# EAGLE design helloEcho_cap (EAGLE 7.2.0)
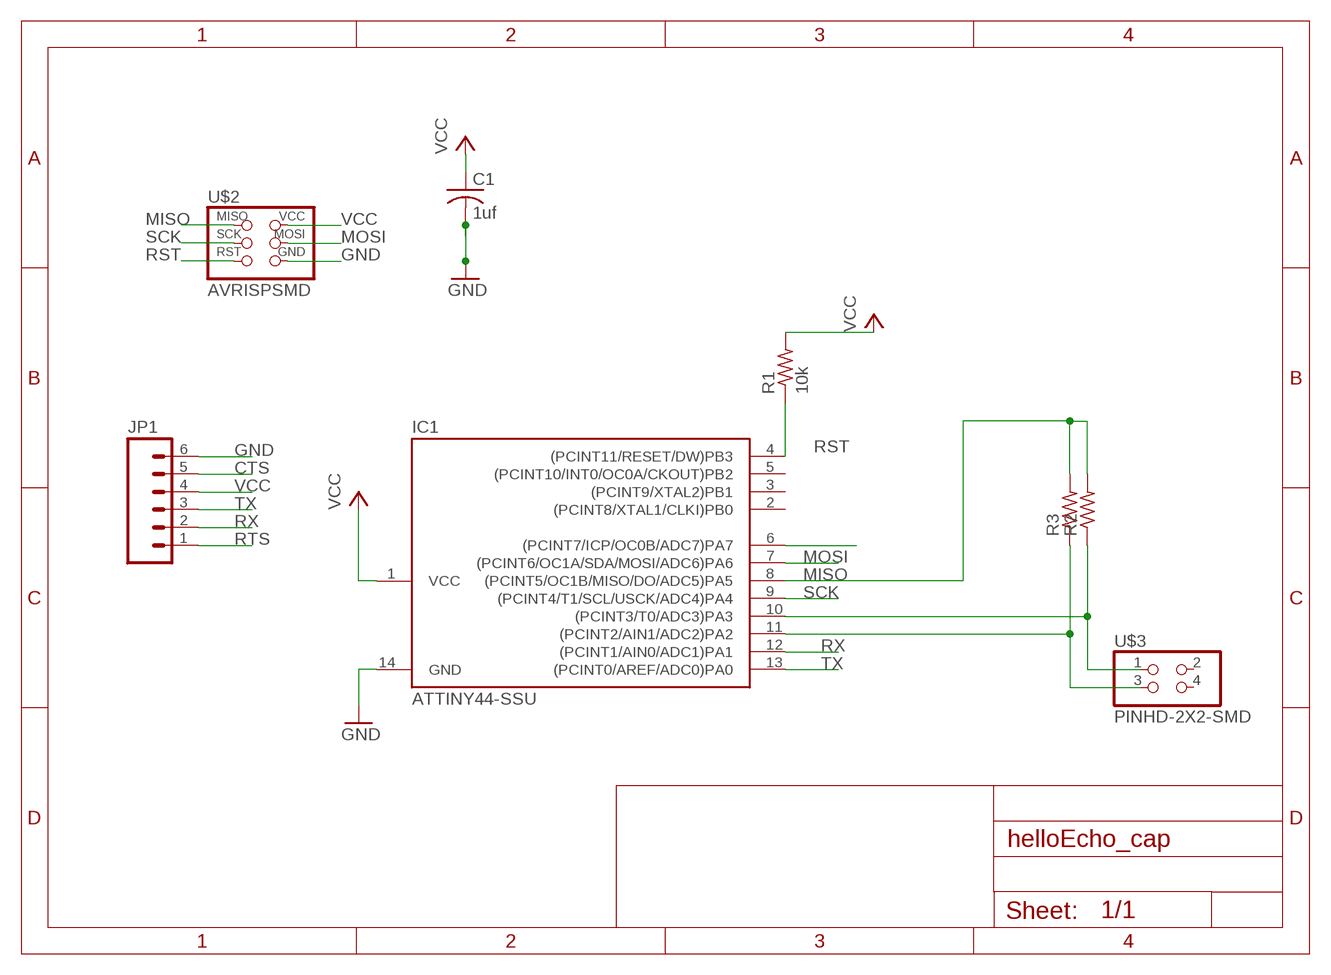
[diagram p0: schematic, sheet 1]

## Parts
C1  1uf  C-USC1206  [C1206]
IC1  ATTINY44-SSU  [SOIC14]
JP1  M06SMD  [1X06-SMD]
R1  10k  R-US_R1206  [R1206]
R2  RESISTOR1206  [1206]
R3  RESISTOR1206  [1206]
U$2  AVRISPSMD  [2X03SMD]
U$3  PINHD-2X2-SMD  [2X02SMD]

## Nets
CTS: JP1.5
GND: C1.2 IC1.14(GND) JP1.6 U$2.6(GND)
MISO: IC1.8((PCINT5/OC1B/MISO/DO/ADC5)PA5) R2.2 R3.2 U$2.1(MISO)
MOSI: IC1.7((PCINT6/OC1A/SDA/MOSI/ADC6)PA6) U$2.4(MOSI)
N$3: IC1.6((PCINT7/ICP/OC0B/ADC7)PA7)
N$5: IC1.10((PCINT3/T0/ADC3)PA3) R2.1 U$3.1
N$6: IC1.11((PCINT2/AIN1/ADC2)PA2) R3.1 U$3.3
RST: IC1.4((PCINT11/RESET/DW)PB3) R1.1 U$2.5(RST)
RTS: JP1.1
RX: IC1.12((PCINT1/AIN0/ADC1)PA1) JP1.2
SCK: IC1.9((PCINT4/T1/SCL/USCK/ADC4)PA4) U$2.3(SCK)
TX: IC1.13((PCINT0/AREF/ADC0)PA0) JP1.3
VCC: C1.1 IC1.1(VCC) JP1.4 R1.2 U$2.2(VCC)
Unconnected: IC1.2((PCINT8/XTAL1/CLKI)PB0) IC1.3((PCINT9/XTAL2)PB1) IC1.5((PCINT10/INT0/OC0A/CKOUT)PB2) U$3.2 U$3.4

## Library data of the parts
C1 = rcl:C-US: CAPACITOR, American symbol
IC1 = fab:ATTINY44
JP1 = SparkFun:M06: Header 6 Standard 6-pin 0.1" header. Use with straight break away headers (SKU : PRT-00116), right angle break away headers (PRT-00553), swiss pins (PRT-00743), machine pins (PRT-00117), and female headers (PRT-00115). Molex polarized connector foot print use with SKU : PRT-08094 with associated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
R1 = resistor:R-US_: RESISTOR, American symbol
R2 R3 = 01_FAB_Hello:RESISTOR
U$2 = fab:AVRISP
U$3 = 01_fab:PINHD-2X2-SMD

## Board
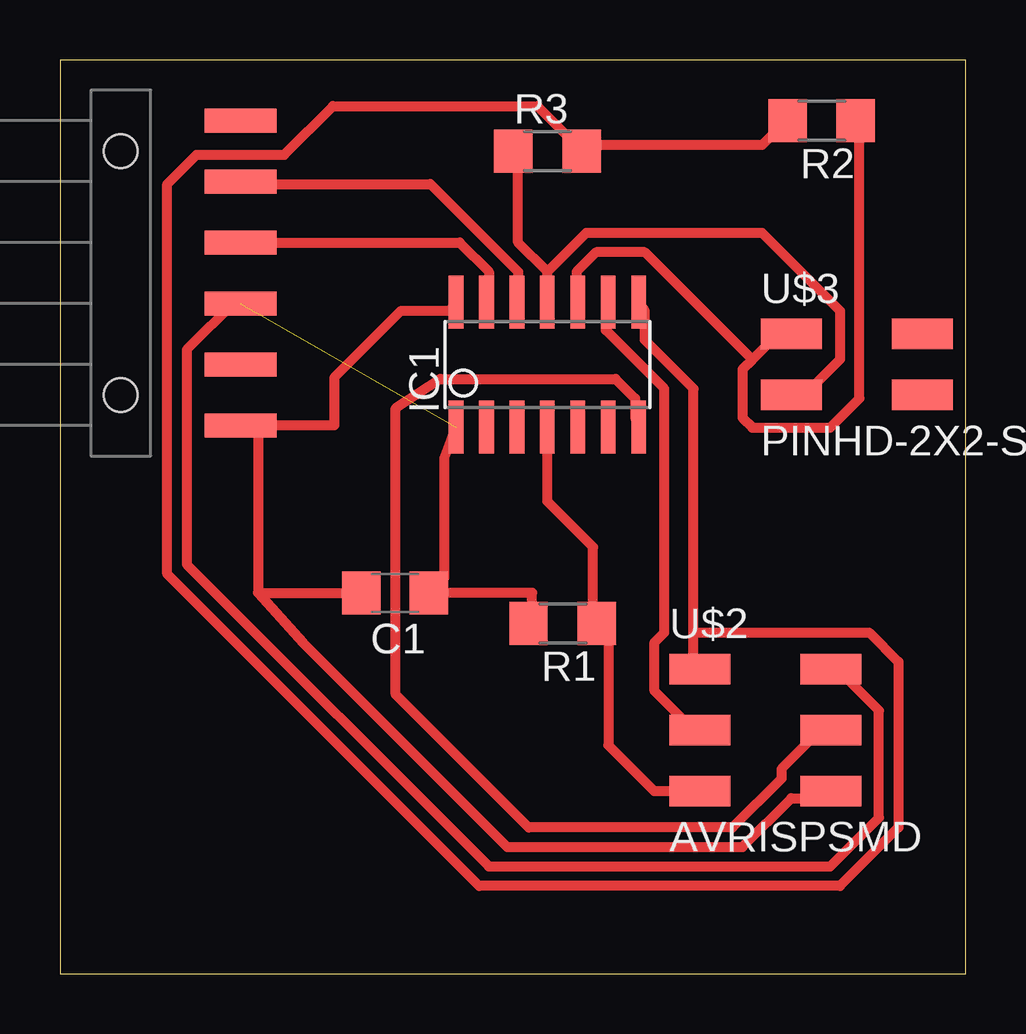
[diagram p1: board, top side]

Size 37.77 x 38.09 mm. Coordinates in mm from the lower left corner, seen from the top.
Outline: 0,0 37.77,0 37.77,38.09 0,38.09 0,0
Copper layers (1*16): Top 0.035mm / dielectric 1.5mm / Bottom 0.035mm
Design rules "default *": minimum track width 16mil, minimum drill 24mil, track to track 16mil, track to pad 16mil, pad to pad 16mil, via to via 16mil, smd to smd 16mil, copper to edge 40mil, drill to drill 8mil, minimum pad ring 10mil, minimum via ring 8mil, stop-mask expansion 4mil, vias tented up to drill 0mil, thermal gap 10mil

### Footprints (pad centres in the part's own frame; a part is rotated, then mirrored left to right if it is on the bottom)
C1206 = smd 1.6 x 1.8: 1 -1.4,0; 2 1.4,0
SOIC14 = smd 0.61 x 2.21: 1 -3.81,-2.603; 2 -2.54,-2.603; 3 -1.27,-2.603; 4 0,-2.603; 5 1.27,-2.603; 6 2.54,-2.603; 7 3.81,-2.603; 8 3.81,2.603; 9 2.54,2.603; 10 1.27,2.603; 11 0,2.603; 12 -1.27,2.603; 13 -2.54,2.603; 14 -3.81,2.603
1X06-SMD = smd 1 x 3: 1 -6.35,5; 2 -3.81,5; 3 -1.27,5; 4 1.27,5; 5 3.81,5; 6 6.35,5 | hole 1.4: -5.08,0; 5.08,0
R1206 = smd 1.6 x 1.803: 1 -1.422,0; 2 1.422,0
1206 = smd 1.6 x 1.803: 1 -1.422,0; 2 1.422,0
2X03SMD = smd 2.54 x 1.27: 1 -2.54,2.54; 2 2.92,2.54; 3 -2.54,0; 4 2.92,0; 5 -2.54,-2.54; 6 2.92,-2.54
2X02SMD = smd 2.54 x 1.27: 1 -2.54,1.27; 2 2.92,1.27; 3 -2.54,-1.27; 4 2.92,-1.27

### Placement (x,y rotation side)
C1  13.97,15.88 180 top
IC1  20.32,25.4 0 top
JP1  2.54,29.21 270 top
R1  20.95,14.61 180 top
R2  31.75,35.56 180 top
R3  20.32,34.29 0 top
U$2  29.21,10.16 0 top
U$3  33.02,25.4 0 top

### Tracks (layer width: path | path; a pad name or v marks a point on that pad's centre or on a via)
GND
  Top 0.406: 7.72,22.76 JP1.6 8.26,22.86 | IC1.14 16.26,27.64 14.22,27.64 11.43,24.84 11.43,22.86 8.26,22.86 | U$2.6 32.11,7.32 30.48,7.32 28.45,5.28 18.64,5.28 10.16,13.77 8.26,15.88 | 8.26,15.88 C1.2 | 8.26,22.86 8.26,15.88
MISO
  Top 0.406: R2.2 30.07,35.36 29.26,34.54 21.95,34.54 R3.2 21.54,34.54 19.91,36.17 11.38,36.17 9.35,34.14 5.69,34.14 4.47,32.92 4.47,16.66 17.48,3.66 32.51,3.66 34.95,6.1 34.95,13.01 33.73,14.22 26.42,14.22 | 26.42,14.22 26.42,13.01 U$2.1 | 26.42,14.22 26.42,24.38 24.38,26.42 24.38,27.64 IC1.8
MOSI
  Top 0.406: U$2.4 31.7,10.16 30.07,8.53 30.07,8.13 28.04,6.1 19.53,6.1 13.99,11.63 13.99,23.57 15.85,24.79 23.16,24.79 23.98,23.98 23.98,23.16 IC1.7
N$5
  Top 0.406: 28.85,25.6 29.67,26.42 30.48,26.42 U$3.1 | 28.85,25.6 28.45,25.2 28.45,23.16 28.85,22.76 32.11,22.76 33.33,23.98 33.33,35.36 R2.1 | 28.85,25.6 24.38,30.07 22.35,30.07 21.54,29.26 21.54,28.04 IC1.10
N$6
  Top 0.406: 20.32,29.26 19.1,30.48 19.1,34.14 R3.1 | IC1.11 20.32,29.26 | 20.32,29.26 21.95,30.89 29.26,30.89 32.51,27.64 32.51,25.6 31.29,24.38 30.48,24.38 U$3.3
RST
  Top 0.406: IC1.4 20.32,19.68 22.23,17.78 22.23,14.76 R1.1 22.86,14.12 22.86,9.53 24.77,7.62 U$2.5
RX
  Top 0.406: IC1.12 19.1,28.04 19.1,29.26 15.44,32.92 7.72,32.92 JP1.2
SCK
  Top 0.406: IC1.9 22.76,27.64 22.76,26.82 25.2,24.38 25.2,14.22 24.79,13.82 24.79,11.79 26.42,10.16 U$2.3
TX
  Top 0.406: JP1.3 16.66,30.48 17.88,29.26 17.88,28.04 IC1.13
VCC  (1 unrouted)
  Top 0.406: IC1.1 16.03,21.49 16.03,16.51 C1.1 19.68,15.88 19.68,14.76 R1.2 | U$2.2 32.51,12.6 34.14,10.97 34.14,6.5 32.11,4.47 17.88,4.47 5.28,17.07 5.28,26.01 7.32,28.04 JP1.4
